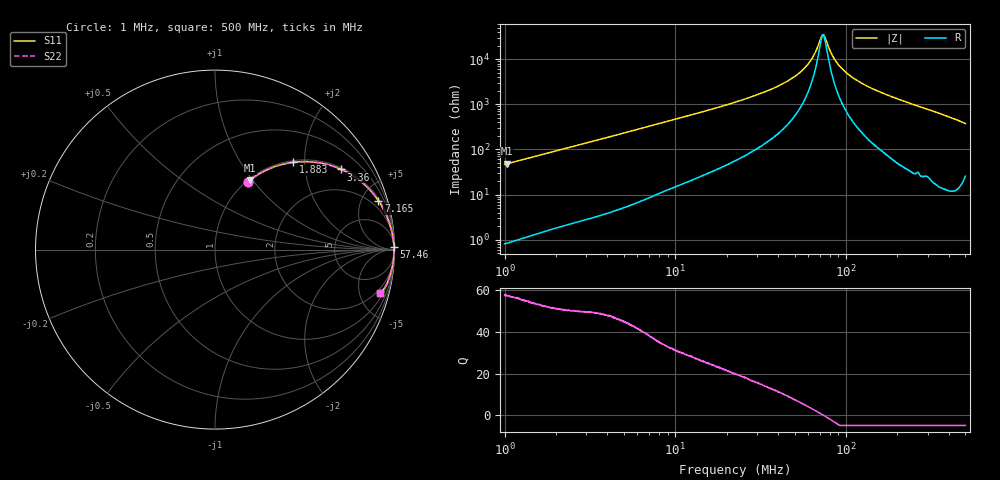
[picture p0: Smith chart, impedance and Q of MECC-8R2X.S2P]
!s-Parameter Generated by FASTRON Sdn. Bhd.
!FASTRON P/N : MECC-8R2X
!Keysight Technologies,E4991B,MY54100416,A.01.15
!Date: Wed Mar 18 10:16:57 2026
!Version  : Rev00 Wed Mar 18 10:16:57 2026
!Data & Calibration Information:
!PortZ  Port1:50+j0  Port2:50+j0
!When reading, reference impedance value at option line is always used.
!Remarks : This data is being provided solely for informational purposes.
!Freq	S11	S21	S12	S22
# Hz S dB R 50
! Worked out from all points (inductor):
!   1601 points, 1 MHz to 500 MHz, reference 50 ohm
!   read as one part in series: L = 7.42 uH near 1.032 MHz
!   highest Q = 57.5 at 1.032 MHz (marker M1), where L = 7.44 uH
!   self-resonance near 73.11 MHz
!   S11 on the Smith chart (normalised r, x): 1 MHz: 1.02, +0.93; 1.883 MHz: 1.03, +1.75; 3.36 MHz: 1.06, +3.11; 7.165 MHz: 1.18, +6.64; 57.46 MHz: open; 500 MHz: 1.51, -7.48
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1000000  -7.52 64.1  -0.92 -24.9  -0.92 -24.9  -7.52 64.1
1031561  -7.30 63.5  -0.97 -25.5  -0.97 -25.5  -7.30 63.5
1883465  -3.71 48.2  -2.55 -40.7  -2.55 -40.7  -3.71 48.2
2820919  -2.09 37.0  -4.41 -51.8  -4.41 -51.8  -2.09 37.0
3359690  -1.58 32.4  -5.41 -56.4  -5.41 -56.4  -1.58 32.4
7165329  -0.44 16.6  -10.86 -71.8  -10.86 -71.8  -0.44 16.6
7957584  -0.37 15.0  -11.71 -73.3  -11.71 -73.3  -0.37 15.0
2.236068e7  -0.07 5.1  -20.99 -82.0  -20.99 -82.0  -0.07 5.1
4.082702e7  -0.04 2.2  -28.46 -82.6  -28.46 -82.6  -0.04 2.2
4.977112e7  -0.03 1.4  -32.25 -81.0  -32.25 -81.0  -0.03 1.4
5.746337e7  -0.03 0.9  -36.27 -77.6  -36.27 -77.6  -0.03 0.9
6.307767e7  -0.03 0.5  -40.26 -71.3  -40.26 -71.3  -0.03 0.5
6.660267e7  -0.03 0.3  -43.62 -63.1  -43.62 -63.1  -0.03 0.3
7.142578e7  -0.03 0.1  -49.59 -29.1  -49.59 -29.1  -0.03 0.1
7.368004e7  -0.02 -0.0  -50.97 6.2  -50.97 6.2  -0.02 -0.0
7.571081e7  -0.02 -0.1  -49.21 34.6  -49.21 34.6  -0.02 -0.1
8.506748e7  -0.03 -0.5  -40.36 72.2  -40.36 72.2  -0.03 -0.5
9.821487e7  -0.03 -1.0  -34.65 80.3  -34.65 80.3  -0.03 -1.0
1.249575e8  -0.03 -2.0  -29.17 83.5  -29.17 83.5  -0.03 -2.0
1.77937e8  -0.04 -3.6  -23.93 83.8  -23.93 83.8  -0.04 -3.6
3.174007e8  -0.11 -7.8  -17.31 80.6  -17.31 80.6  -0.11 -7.8
5e8  -0.44 -14.6  -11.93 71.4  -11.93 71.4  -0.44 -14.6
